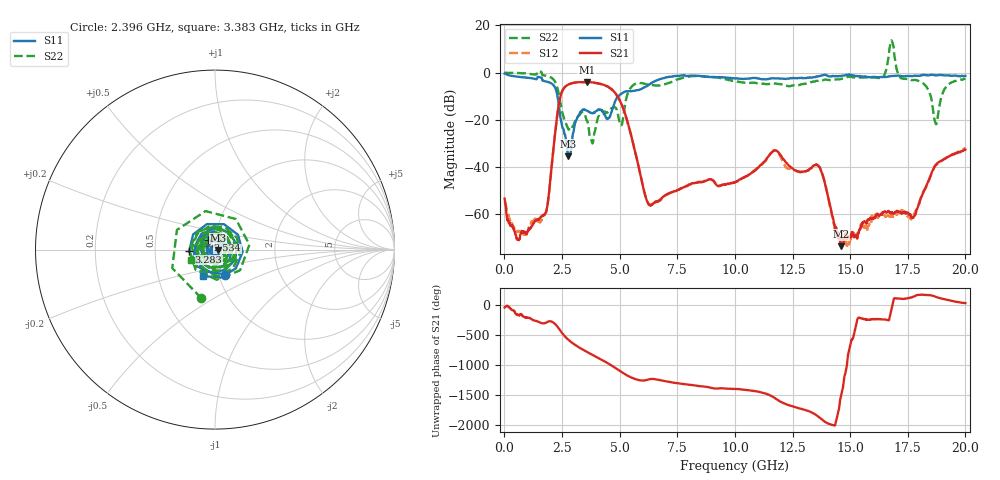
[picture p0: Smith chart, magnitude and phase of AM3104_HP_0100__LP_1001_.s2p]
!Created with skrf (http://scikit-rf.org).
# Hz S RI R 50.0
!freq ReS11 ImS11 ReS21 ImS21 ReS12 ImS12 ReS22 ImS22
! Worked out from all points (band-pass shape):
!   1601 points, 10 MHz to 20 GHz, reference 50 ohm
!   highest |S21| = -3.97 dB at 3.571 GHz (marker M1); lowest = -73.5 dB at 14.6 GHz (marker M2)
!   |S21| within 3 dB of the highest: 2.554 GHz to 4.651 GHz (2.097 GHz wide, 58.2 % of centre)
!   lowest |S11| = -35.4 dB at 2.771 GHz (marker M3), VSWR 1.03, Z = 51.7 - j0.161 ohm
!   |S11| at or under -10 dB: 2.304 GHz to 4.941 GHz (2.637 GHz wide, 72.8 % of centre)
!   |S22| runs from -30.0 to 13.6 dB; largest |S21 - S12| = 0.049
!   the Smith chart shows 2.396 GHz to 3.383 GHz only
!   S11 on the Smith chart (normalised r, x): 2.396 GHz: 1.08, -0.31; 2.534 GHz: 0.92, +0.10; 3.283 GHz: 0.75, -0.02; 3.383 GHz: 0.84, -0.26
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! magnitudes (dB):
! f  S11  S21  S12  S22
! 10 MHz  -0.4  -53.4  -54.9  0.0
! 572.2 MHz  -1.7  -70.9  -67.1  -0.1
! 1.709 GHz  -3.5  -60.5  -60.2  -1.1
! 2.396 GHz  -16.5  -11.7  -11.7  -11.0
! 2.534 GHz  -23.6  -7.3  -7.3  -17.6
! 2.771 GHz  -35.4  -5.0  -5.1  -24.0
! 3.283 GHz  -16.8  -4.0  -4.1  -17.6
! 3.346 GHz  -16.2  -4.0  -4.1  -16.8
! 3.383 GHz  -15.8  -4.0  -4.1  -16.9
! 3.571 GHz  -16.1  -4.0  -4.1  -20.2
! 3.796 GHz  -17.1  -4.1  -4.1  -29.3
! 4.908 GHz  -10.4  -10.0  -10.1  -16.6
! 6.182 GHz  -5.7  -54.3  -54.4  -5.0
! 6.682 GHz  -3.0  -54.5  -54.4  -5.5
! 10.01 GHz  -2.5  -46.6  -46.4  -3.7
! 11.72 GHz  -2.4  -33.0  -33.1  -4.6
! 13.34 GHz  -2.1  -40.2  -40.2  -4.0
! 14.6 GHz  -1.4  -73.5  -70.3  -2.7
! 16.68 GHz  -1.6  -58.9  -60.9  7.2
! 17.75 GHz  -1.3  -61.3  -60.8  -3.1
! 18.71 GHz  -1.2  -39.0  -39.4  -21.6
! 20 GHz  -1.4  -32.6  -32.0  -2.6
